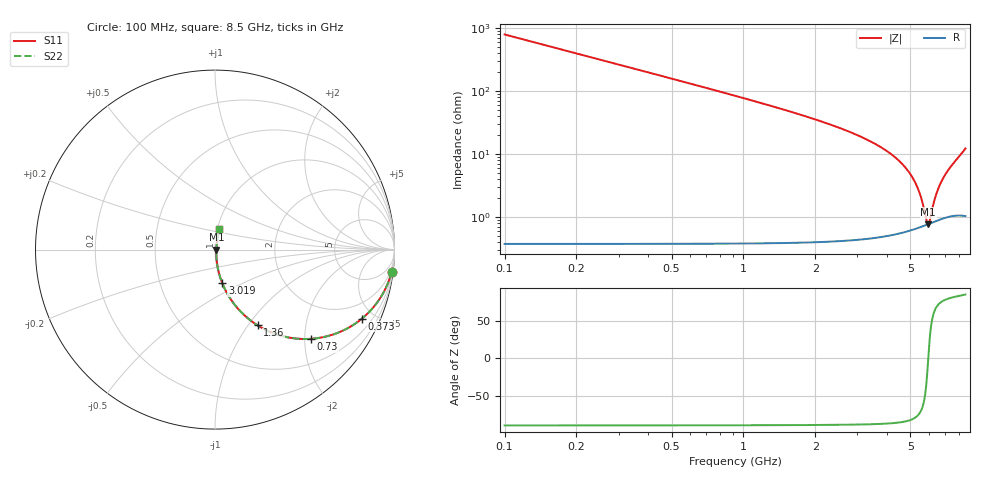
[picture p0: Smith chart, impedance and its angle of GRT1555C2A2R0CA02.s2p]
!Murata Part Number: GRT1555C2A2R0CA02
!These Parameters are Measured in Series Mode Connection
!Data Generated on Jun 19, 2026
!  o--ll--o
!Port1  Port2
!  o------o
!Operation Temp=25[degC], DC Bias Voltage=0[V]
!Freq. Start=100[MHz] Stop=9[GHz] 401[Steps]
# Hz S RI R 50
!Freq.(Hz) S11(Real) S11(Imag) S21(Real) S21(Imag) S12(Real) S12(Imag) S22(Real) S22(Imag)
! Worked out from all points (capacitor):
!   401 points, 100 MHz to 8.5 GHz, reference 50 ohm
!   read as one part in series: C = 2 pF near 142 MHz
!   lowest |Z| = 763 mohm at 5.938 GHz (marker M1)
!   series resonance near 5.943 GHz, so ESL is about 360 pH
!   S11 on the Smith chart (normalised r, x): 100 MHz: 1, -16; 373 MHz: 1.01, -4.25; 730 MHz: 1.01, -2.15; 1.36 GHz: 1.01, -1.11; 3.019 GHz: 1.01, -0.39; 8.5 GHz: 1.02, +0.24
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1e8  0.9844 -0.1237  0.0156 0.1237  0.0156 0.1237  0.9844 -0.1237
2.26e8  0.9249 -0.263  0.0751 0.263  0.0751 0.263  0.9249 -0.263
3.73e8  0.8183 -0.3847  0.1817 0.3847  0.1817 0.3847  0.8183 -0.3847
7.3e8  0.5355 -0.497  0.4645 0.497  0.4645 0.497  0.5355 -0.497
1.024e9  0.3635 -0.4785  0.6365 0.4785  0.6365 0.4785  0.3635 -0.4785
1.36e9  0.2372 -0.4219  0.7628 0.4219  0.7628 0.4219  0.2372 -0.4219
1.507e9  0.1986 -0.3951  0.8014 0.3951  0.8014 0.3951  0.1986 -0.3951
2.095e9  0.103 -0.2981  0.897 0.2981  0.897 0.2981  0.103 -0.2981
2.914e9  0.0454 -0.1983  0.9546 0.1983  0.9546 0.1983  0.0454 -0.1983
3.019e9  0.0411 -0.1879  0.9589 0.1879  0.9589 0.1879  0.0411 -0.1879
4.3e9  0.013 -0.0877  0.987 0.0877  0.987 0.0877  0.013 -0.0877
4.804e9  0.00908 -0.0575  0.9909 0.0575  0.9909 0.0575  0.00908 -0.0575
5.182e9  0.00765 -0.037  0.9924 0.037  0.9924 0.037  0.00765 -0.037
5.476e9  0.00723 -0.0221  0.9928 0.0221  0.9928 0.0221  0.00723 -0.0221
5.707e9  0.00726 -0.0109  0.9927 0.0109  0.9927 0.0109  0.00726 -0.0109
5.854e9  0.00742 -0.00408  0.9926 0.00408  0.9926 0.00408  0.00742 -0.00408
5.938e9  0.00756 -0.000237  0.9924 0.000237  0.9924 0.000237  0.00756 -0.000237
6.022e9  0.00774 0.00356  0.9923 -0.00356  0.9923 -0.00356  0.00774 0.00356
6.274e9  0.00843 0.0147  0.9916 -0.0147  0.9916 -0.0147  0.00843 0.0147
6.484e9  0.00918 0.0237  0.9908 -0.0237  0.9908 -0.0237  0.00918 0.0237
7.114e9  0.0122 0.0496  0.9878 -0.0496  0.9878 -0.0496  0.0122 0.0496
8.5e9  0.0243 0.1174  0.9757 -0.1174  0.9757 -0.1174  0.0243 0.1174
